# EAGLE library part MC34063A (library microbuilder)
MC34063A - 1.5A 3V-40V Boost/Buck/Inverting Voltage Regulator [Part No.] Allows you to 'boost', reduce or invert the voltage of your power supply to a more appropriate level. Common voltage regulators like the LM1117 are easy to use, but they can only 'reduce' the voltage level and require more volts than they provide, making them useless for low voltage power supplies like batteries or solar panels. A 'Step-Up' regulator like the MC34063A solves this problem by also allowing you to increase the voltage to a pre-determined level, though you still need to pay attention to the minimum voltage level the converter can handle, keeping in mind that many 'step-up' converts are less efficient at the two extreme ends of their working range. Given that many step-up circuits introduce some ripple to the power supply, you can often get a much 'smoother' supply by boosting the voltage up to 5.0V and then using a standard fixed voltage regulator (such as the common LM1117, etc.) to drop the voltage back down to 3.3V. This may not be necessary, and some step up regulators can provide a smooth supply on their own, but it's worth keeping in mind if you do encounter some ripple in the power supply using only a step-up IC for your power supply. Texas Instruments MC34063A Digikey: 296-17765-1-ND
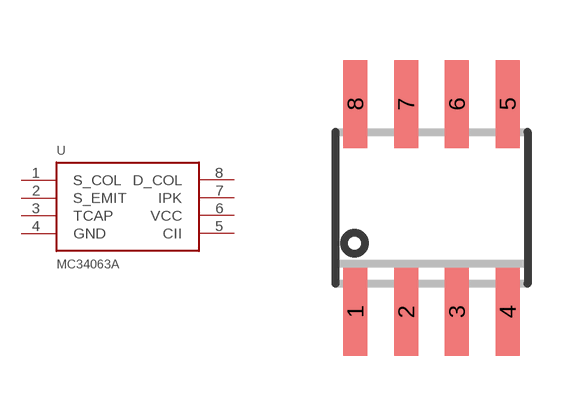
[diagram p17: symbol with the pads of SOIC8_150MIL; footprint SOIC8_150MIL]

Designator prefix U

## MC34063A  [SOIC8_150MIL]
1  S_COL
2  S_EMIT
3  TCAP
4  GND
5  CII
6  VCC
7  IPK
8  D_COL

## Footprint SOIC8_150MIL (pad centres in mm)
Small Outline IC - 150mil Wide
smd 0.6 x 2.2: 1 -1.905,-2.6; 2 -0.635,-2.6; 3 0.635,-2.6; 4 1.905,-2.6; 5 1.905,2.6; 6 0.635,2.6; 7 -0.635,2.6; 8 -1.905,2.6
